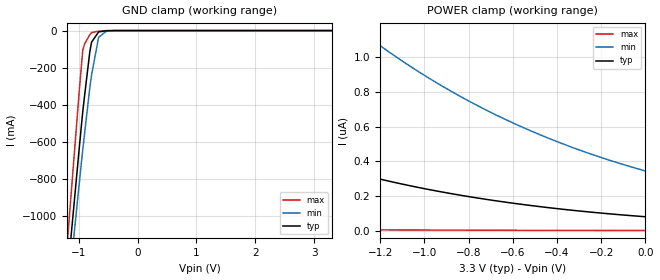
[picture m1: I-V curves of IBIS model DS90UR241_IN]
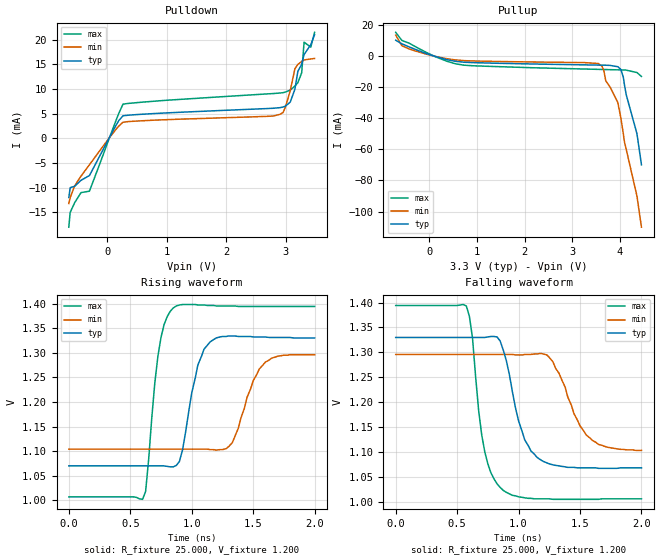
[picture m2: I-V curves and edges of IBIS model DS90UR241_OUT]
|   National Semiconductor Corporation
|   Displays Product Group
|   IBIS Model of DS90UR241IVS
|   48 TQFP
[IBIS Ver]   3.2
[Comment char]  |_char
[File name]   ds90ur241ivs.ibs
[File Rev]   1.0
[Date]   11/16/2006
[Source]   Simulation based model
[Notes]
IBIS Parser Results:
Checking ds90ur241ivs.ibs for IBIS 3.2 Compatibility...
Errors  : 0
File Passed
* Rev 1.0 Comments:
- Revision date: 11/16/06
- Revision 1.0: The original model
Model Comments:
Created by cdytsc
* END Rev 1.0 Comments
[Disclaimer]
(C) Copyright National Semiconductor Corporation 2006
   All rights reserved
   National Semiconductor Corporation hereby grants
the user of this IBIS model a non-exclusive, nontransferable
license to use this IBIS model under the following terms.
Before using this IBIS model, the user should read this
license.  If the user does not accept these terms,  the
IBIS model should be returned to National within 30 days.
   The user is granted this license only to use the
IBIS model and is not granted rights to sell, load, rent,
lease or license the IBIS model in whole or in part, or in
modified form to anyone other than user. User may modify
the IBIS model to suit its specific applications but rights
to derivative works and such modifications shall belong to
National.
   This IBIS model is provided on an "AS IS" basis and
National makes absolutely no warranty with respect to the
information contained herein.NATIONAL DISCLAIMS AND CUSTOMER
WAIVES ALL WARRANTIES, EXPRESS OR IMPLIED, INCLUDING
WARRANTIES OF MERCHANTABILITY OR FITNESS FOR A PARTICULAR
PURPOSE. The entire risk as to quality and performance is
with the Customer. ACCORDINGLY, IN NO EVENT SHALL THE
COMPANY BE LIABLE FOR ANY DAMAGES, WHETHER IN CONTRACT OR
TORT,INCLUDING ANY LOST PROFITS OR OTHER INCIDENTAL,
CONSEQUENTIAL, EXEMPLARY, OR PUNITIVE DAMAGES ARISING OUT
OF THE USE OR APPLICATION OF THE IBIS model provided in
this package.Further, National reserves the right to make
changes without notice to any product herein to improve
reliability, function, or design. National does not convey
any license under patent rights or any other intellectual
property rights, including those of third parties.
   National is not obligated to provide maintenance or support
for the licensed IBIS model.
Contact National at ATTN:DISPLAYS APPLICATIONS/IBIS MODELS.
2900 Semiconductor Drive, M/S A2595, Santa Clara, CA 95052-8090
[Copyright]   Copyright 2006, National Semiconductor, All Rights Reserved
[Component]   DS90UR241IVS
[Manufacturer]  National Semiconductor Corp
[Package]
|   typ   min   max
R_pkg   0.134   0.117   0.164
L_pkg   3.430nH   3.040nH   4.129nH
C_pkg   0.183pF   0.159pF   0.229pF
[Pin]   signal_name  model_name   R_pin   L_pin   C_pin
1   DIN20   DS90UR241_IN   0.157   4.129n   0.209p
2   DIN21   DS90UR241_IN   0.164   3.756n   0.170p
3   DIN22   DS90UR241_IN   0.147   3.458n   0.160p
4   DIN23   DS90UR241_IN   0.133   3.221n   0.159p
5   RESVRD   NC   0.124   3.048n   0.162p
6   VSSL   GND   0.117   3.040n   0.229p
7   VDDL   POWER   0.120   3.040n   0.229p
8   RESVRD   NC   0.117   3.048n   0.162p
9   TPWDNB   DS90UR241_IN   0.124   3.221n   0.159p
10   TCLK   DS90UR241_IN   0.133   3.458n   0.160p
11   TRFB   DS90UR241_IN   0.147   3.756n   0.170p
12   RAOFF   DS90UR241_IN   0.164   4.129n   0.209p
13   RESVRD   NC   0.157   3.959n   0.206p
14   VDDPT1   POWER   0.143   3.678n   0.182p
15   VSSPT1   GND   0.133   3.448n   0.169p
16   VDDPT0   POWER   0.125   3.256n   0.167p
17   VSSPT0   GND   0.119   3.110n   0.176p
18   DEN   DS90UR241_IN   0.120   3.062n   0.210p
19   DOUTM   DS90UR241_OUT   0.120   3.062n   0.210p
20   DOUTP   DS90UR241_OUT   0.119   3.110n   0.176p
21   VSSDR   GND   0.125   3.256n   0.167p
22   VDDDR   POWER   0.133   3.448n   0.169p
23   PRE   DS90UR241_IN   0.143   3.678n   0.182p
24   RESVRD   NC   0.157   3.959n   0.206p
25   DIN0   DS90UR241_IN   0.164   4.129n   0.209p
26   DIN1   DS90UR241_IN   0.147   3.756n   0.170p
27   DIN2   DS90UR241_IN   0.133   3.458n   0.160p
28   DIN3   DS90UR241_IN   0.124   3.221n   0.159p
29   DIN4   DS90UR241_IN   0.117   3.048n   0.162p
30   VDDT   GND   0.120   3.040n   0.229p
31   VSST   POWER   0.120   3.040n   0.229p
32   DIN5   DS90UR241_IN   0.117   3.048n   0.162p
33   DIN6   DS90UR241_IN   0.124   3.221n   0.159p
34   DIN7   DS90UR241_IN   0.133   3.458n   0.160p
35   DIN8   DS90UR241_IN   0.147   3.756n   0.170p
36   DIN9   DS90UR241_IN   0.164   4.129n   0.209p
37   DIN10   DS90UR241_IN   0.157   3.959n   0.206p
38   DIN11   DS90UR241_IN   0.143   3.678n   0.182p
39   DIN12   DS90UR241_IN   0.133   3.448n   0.169p
40   DIN13   DS90UR241_IN   0.125   3.256n   0.167p
41   DIN14   DS90UR241_IN   0.119   3.110n   0.176p
42   VDDT   POWER   0.120   3.062n   0.210p
43   VSST   GND   0.120   3.062n   0.210p
44   DIN15   DS90UR241_IN   0.119   3.110n   0.176p
45   DIN16   DS90UR241_IN   0.125   3.256n   0.167p
46   DIN17   DS90UR241_IN   0.133   3.448n   0.169p
47   DIN18   DS90UR241_IN   0.143   3.678n   0.182p
48   DIN19   DS90UR241_IN   0.157   3.959n   0.206p
[Diff_pin]   inv_pin   vdiff   tdelay_typ   tdelay_min   tdelay_max
| The '+' pin is Diff_pin and the '-' pin is the inv_pin
20   19   0.05   0   0   0
| Models and submodels in the file (2): DS90UR241_IN (Input), DS90UR241_OUT (3-state)
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|   TTL INPUT PINS MODEL
[Model]   DS90UR241_IN
Model_type   Input
Vinh=2.0
Vinl=0.8
|   typ   min   max
C_comp   1.535pF   1.314pF   1.827pF
|   typ   min   max
[Temperature Range]   25.0   105.0   -40.0
[Voltage range]   3.3V   3.0V   3.6V
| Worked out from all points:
|   GND clamp passes 1 mA (typ) near -0.53 V on its own axis
[Power_clamp]
| Note that the [POWER_clamp] voltage table is referenced to Vcc
| and is calculated using Vtable = Vcc - Vmeasured.
|Voltage   I(typ)   I(min)   I(max)
-3.3V     1.955uA    5.164uA    48.51nA
-2.67V    1.159uA    3.356uA    24.24nA
-2.37V    893.1nA    2.702uA    17.21nA
-2.19V    761nA      2.364uA    13.97nA
-2.04V    664.2nA    2.109uA    11.71nA
-1.86V    562.7nA    1.834uA    9.446nA
-1.65V    461.4nA    1.551uA    7.319nA
-1.29V    324.9nA    1.152uA    4.68nA
-990mV    239.4nA    887.1nA    3.182nA
-660mV    168.8nA    657nA      2.057nA
-330mV    117.1nA    479.1nA    1.31nA
0V        79.92nA    343.7nA    822.8pA
[GND_clamp]
|Voltage   I(typ)   I(min)   I(max)
|VCC   3.3   3   3.6
|Temp   25C   105   -40C
|   Typ   Min   Max
-3.3V     -8.95A     -8.398A    -10.31A
-1.2V     -1.361A    -1.489A    -1.183A
-990mV    -640.9mA   -831.2mA   -333.4mA
-930mV    -441.4mA   -647.4mA   -109.6mA
-900mV    -357.3mA   -562.2mA   -73.49mA
-810mV    -116.7mA   -311.7mA   -22.18mA
-780mV    -63.01mA   -241.1mA   -11.12mA
-660mV    -7.352mA   -36.56mA   -3.142mA
-540mV    -1.31mA    -6.06mA    -523uA
-510mV    -614.8uA   -2.617mA   -226.3uA
3.3V      1.602nA    13.71nA    15.32pA
|   0% Pre-emphasis LVDS OUTPUT PINS MODEL
[Model]   DS90UR241_OUT
Model_type 3-state
Enable Active-High
Polarity Inverting
Vref=1.2
Vmeas=1.2
Rref=50   | two 100 Ohms Across Outputs DOUTP and DOUTM
Cref=5p
C_comp   2pF   2pF   2pF
[Temperature Range]   25.0   105.0   -40.0
[Voltage range]   3.3V   3.0V   3.6V
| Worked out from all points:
|   slope of the pulldown table from 0 to 0.495 V, typ, clamps not added: 89.3 ohm
|   slope of the pullup table from 0 to 0.495 V, typ, clamps not added: 122 ohm
|   falling waveform, R_fixture 25.000, V_fixture 1.200: 20-80 % time 154ps typ, 201ps min, 113ps max; typ from 1.33 V to 1.07 V
|   rising waveform, R_fixture 25.000, V_fixture 1.200: 20-80 % time 116ps typ, 161ps min, 90.4ps max; typ from 1.07 V to 1.33 V
[Pullup]
|Vtable   I(typ)   I(min)   I(max)
-699mV    9.96mA     13.2mA     15mA
-570mV    7.63mA     6.44mA     9.8mA
-419mV    5.67mA     4.34mA     8.04mA
556mV     -3.61mA    -2.72mA    -5.21mA
3.622V    -6.06mA    -6.74mA    -8.82mA
3.702V    -6.11mA    -16.2mA    -8.88mA
3.953V    -7.05mA    -30mA      -9.07mA
4.018V    -8.78mA    -40mA      -9.12mA
4.091V    -18.4mA    -55mA      -9.19mA
4.129V    -25mA      -60mA      -9.25mA
4.354V    -50mA      -90mA      -10.8mA
4.449V    -70mA      -110mA     -13.3mA
[Pulldown]
|V(pulldown)   I(typ)   I(min)   I(max)
-643mV    -12mA      -13.2mA    -18mA
-620mV    -10mA      -12mA      -15mA
-438mV    -8.5mA     -7.66mA    -11mA
-296mV    -7.53mA    -5.34mA    -10.7mA
268mV     4.58mA     3.27mA     6.94mA
2.8V      6.11mA     4.54mA     9.09mA
3V        6.55mA     6.38mA     9.4mA
3.158V    9.96mA     14.1mA     10.6mA
3.272V    15mA       15.6mA     13.3mA
3.313V    17mA       15.9mA     19.5mA
3.425V    19mA       16.1mA     18.5mA
3.489V    21mA       16.2mA     21.5mA
[Ramp]
dV/dt_r   0.1572/.1144ns   0.1275/.1589ns   0.2248/.0889ns
dV/dt_f   0.1571/.1503ns   0.1263/.2010ns   0.2247/.1119ns
R_load=50
[Falling Waveform]
R_fixture = 25.000
V_fixture = 1.200
|  time   V(typ)   V(min)   V(max)
0s        1.33V      1.296V     1.394V
575ps     1.33V      1.296V     1.393V
625ps     1.33V      1.296V     1.329V
725ps     1.33V      1.296V     1.101V
875ps     1.305V     1.296V     1.024V
1ns       1.163V     1.295V     1.011V
1.15ns    1.09V      1.297V     1.007V
1.28ns    1.075V     1.281V     1.006V
1.55ns    1.069V     1.135V     1.006V
2ns       1.069V     1.104V     1.007V
[Rising Waveform]
R_fixture = 25.000
V_fixture = 1.200
|  time   V(typ)   V(min)   V(max)
0s        1.07V      1.104V     1.007V
600ps     1.07V      1.104V     1.002V
625ps     1.07V      1.104V     1.018V
725ps     1.07V      1.104V     1.293V
850ps     1.068V     1.104V     1.391V
1.05ns    1.275V     1.104V     1.397V
1.15ns    1.322V     1.103V     1.396V
1.33ns    1.334V     1.117V     1.395V
1.6ns     1.332V     1.281V     1.394V
2ns       1.33V      1.296V     1.394V
